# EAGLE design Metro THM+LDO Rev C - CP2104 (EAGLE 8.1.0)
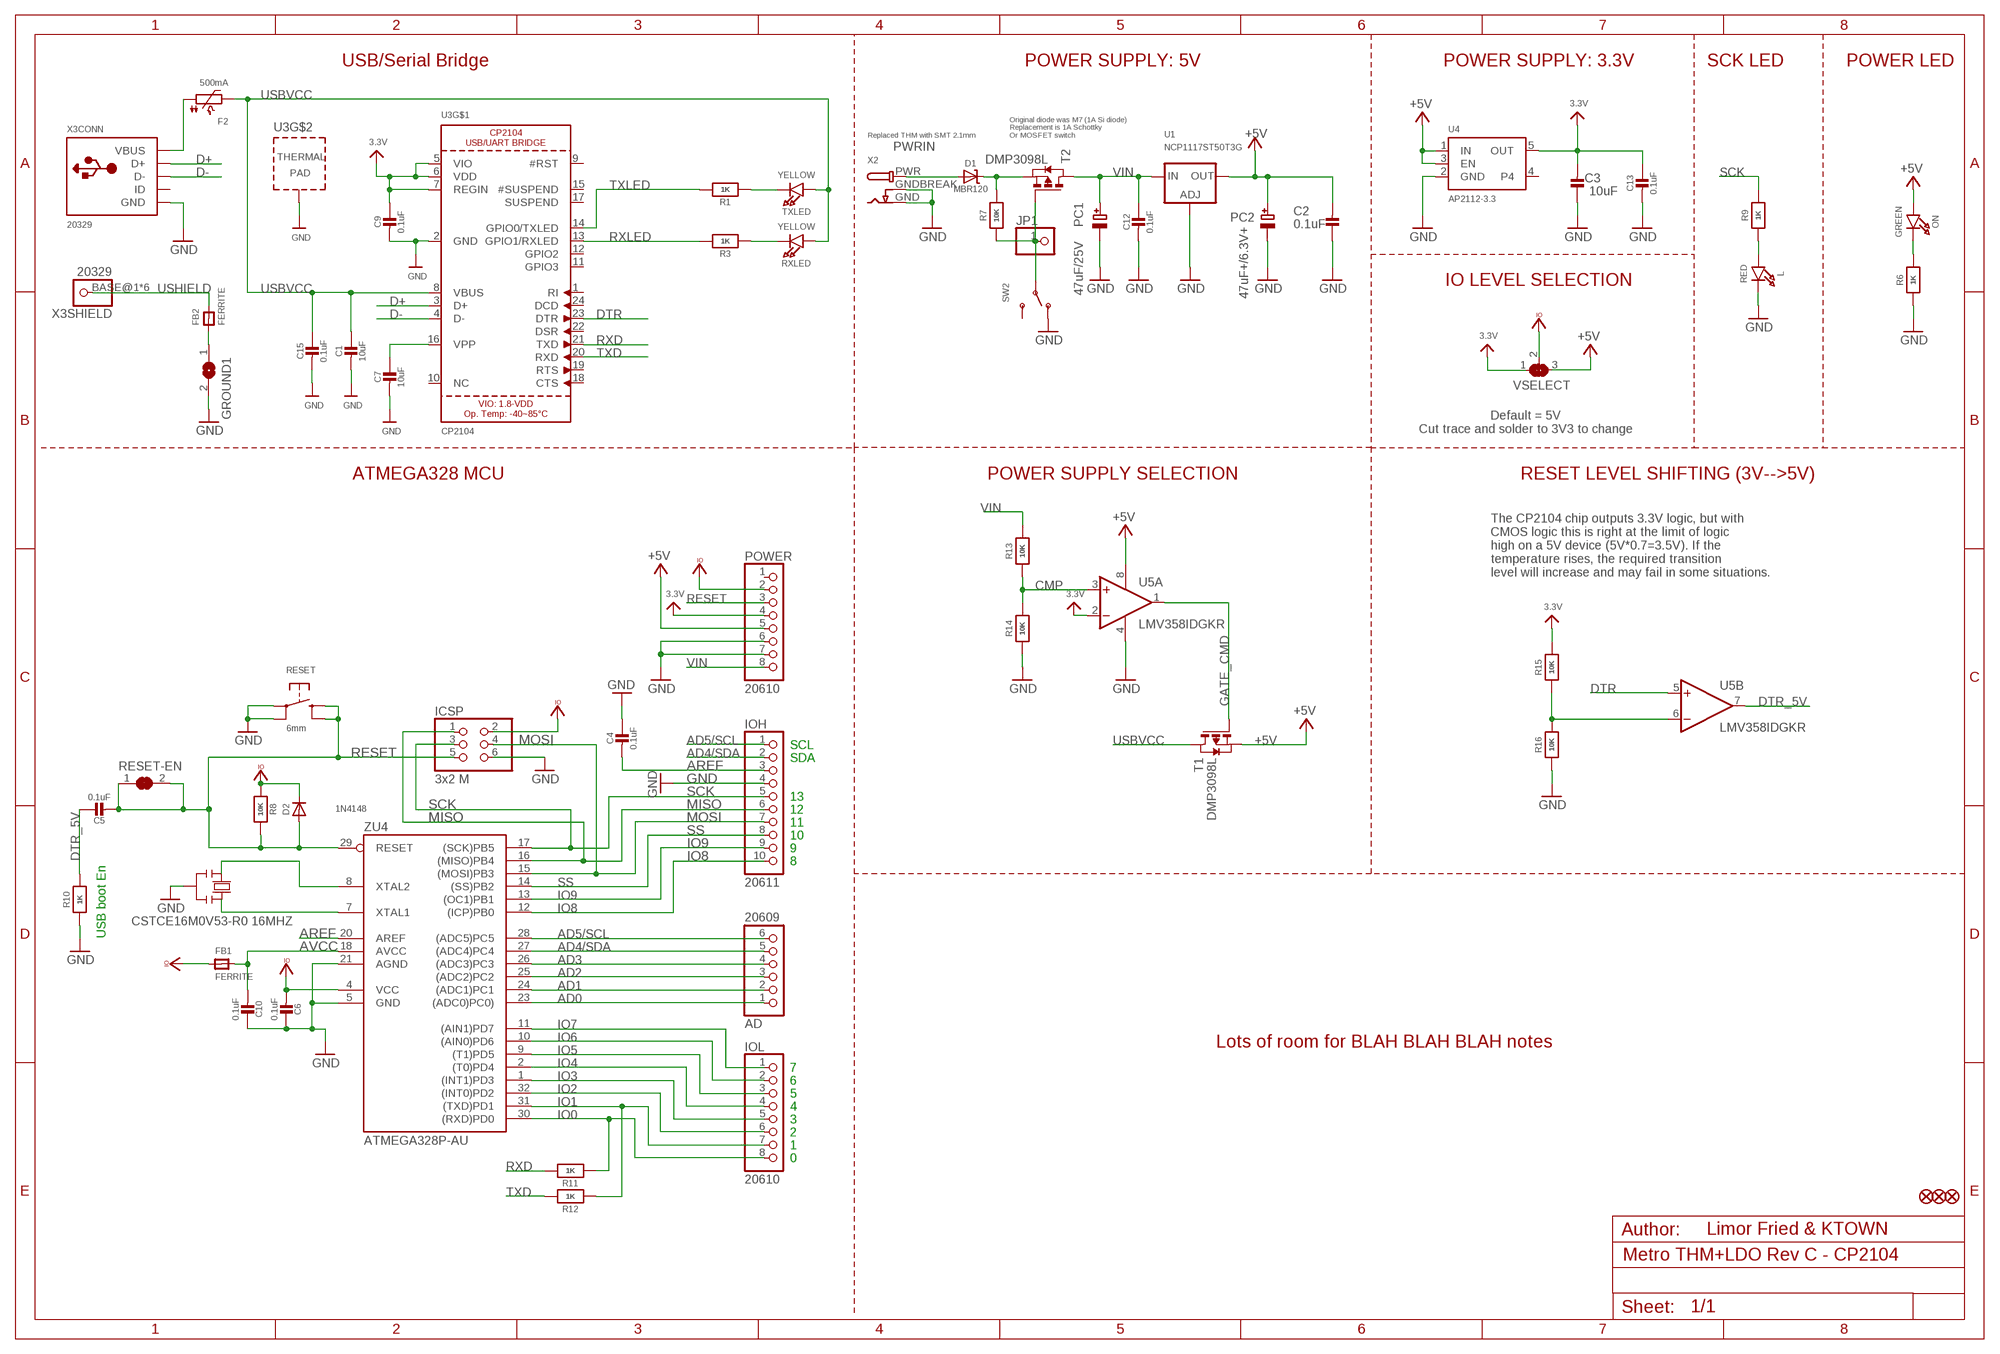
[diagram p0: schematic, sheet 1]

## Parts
AD  20609  HEADER-1X6  [1X06_OVAL]
C1  10uF  CAP_CERAMIC0805-NOOUTLINE  [0805-NO]
C2  0.1uF  CAP_CERAMIC0805-NOOUTLINE  [0805-NO]
C3  10uF  CAP_CERAMIC0805-NOOUTLINE  [0805-NO]
C4  0.1uF  CAP_CERAMIC0805-NOOUTLINE  [0805-NO]
C5  0.1uF  CAP_CERAMIC0805-NOOUTLINE  [0805-NO]
C6  0.1uF  CAP_CERAMIC0805-NOOUTLINE  [0805-NO]
C7  10uF  CAP_CERAMIC0805-NOOUTLINE  [0805-NO]
C9  0.1uF  CAP_CERAMIC0805-NOOUTLINE  [0805-NO]
C10  0.1uF  CAP_CERAMIC0805_10MGAP  [0805_10MGAP]
C12  0.1uF  CAP_CERAMIC0805-NOOUTLINE  [0805-NO]
C13  0.1uF  CAP_CERAMIC0805-NOOUTLINE  [0805-NO]
C15  0.1uF  CAP_CERAMIC0805-NOOUTLINE  [0805-NO]
D1  MBR120  DIODE-SCHOTTKYSOD-123  [SOD-123]
D2  1N4148  DIODESOD-323  [SOD-323]
F2  500mA  PTC_1206NO  [1206-NO]
FB1  FERRITE  FERRITE-0805NO  [0805-NO]
FB2  FERRITE  FERRITE-0805NO  [0805-NO]
FD1  FIDUCIAL_1MM  [FIDUCIAL_1MM]
FD2  FIDUCIAL_1MM  [FIDUCIAL_1MM]
FD3  FIDUCIAL_1MM  [FIDUCIAL_1MM]
GROUND1  SJ  [SJ]
ICSP  3x2 M  HEADER-2X3  [2X03_ROUND_70MIL]
IOH  20611  HEADER-1X10  [1X10_OVAL]
IOL  20610  HEADER-1X8  [1X08_OVAL]
JP1  HEADER-1X1ROUND  [1X01_ROUND]
L  RED  LED0805_NOOUTLINE  [CHIPLED_0805_NOOUTLINE]
ON  GREEN  LED0805_NOOUTLINE  [CHIPLED_0805_NOOUTLINE]
PC1  47uF/25V  CAP_ELECTROLYTICPANASONIC_D  [PANASONIC_D]
PC2  47uF+/6.3V+  CAP_ELECTROLYTICPANASONIC_D  [PANASONIC_D]
POWER  20610  HEADER-1X8  [1X08_OVAL]
R1  1K  RESISTOR0805_NOOUTLINE  [0805-NO]
R3  1K  RESISTOR0805_NOOUTLINE  [0805-NO]
R6  1K  RESISTOR0805_NOOUTLINE  [0805-NO]
R7  10K  RESISTOR0805_NOOUTLINE  [0805-NO]
R8  10K  RESISTOR_0805MP  [_0805MP]
R9  1K  RESISTOR0805_NOOUTLINE  [0805-NO]
R10  1K  RESISTOR0805_NOOUTLINE  [0805-NO]
R11  1K  RESISTOR0805_NOOUTLINE  [0805-NO]
R12  1K  RESISTOR0805_NOOUTLINE  [0805-NO]
R13  10K  RESISTOR0805_NOOUTLINE  [0805-NO]
R14  10K  RESISTOR0805_NOOUTLINE  [0805-NO]
R15  10K  RESISTOR0805_NOOUTLINE  [0805-NO]
R16  10K  RESISTOR0805_NOOUTLINE  [0805-NO]
RESET  6mm  SWITCH_TACT_SMT  [EVQ-Q2]
RESET-EN  SOLDERJUMPER_CLOSED  [SOLDERJUMPER_CLOSEDWIRE]
RXLED  YELLOW  LED0805_NOOUTLINE  [CHIPLED_0805_NOOUTLINE]
SW2  SWITCH_SPDT  [SPDT_SMT_SSSS811101]
T1  DMP3098L  PMOSSOT23  [SOT-23]
T2  DMP3098L  PMOSSOT23  [SOT-23]
TXLED  YELLOW  LED0805_NOOUTLINE  [CHIPLED_0805_NOOUTLINE]
U1  NCP1117ST50T3G  LM1117SOT223-REFLOW  [SOT223-R]
U3  CP2104  [QFN24_4MM_SMSC]
U4  AP2112-3.3  VREG_SOT23-5  [SOT23-5]
U5  LMV358IDGKR  LMV358MMX  [MSOP08]
VSELECT  SOLDERJUMPER_2WAY  [SOLDERJUMPER_2WAY_OPEN_NOPASTE]
X2  DCBARRELPTH  [DCJACK_2MM_PTH]
X3  20329  USB_W_SHIELD_V2  [4UCONN_20329_V2]
Y2  CSTCE16M0V53-R0 16MHZ  RESONATORMU  [RESONATOR]
ZU4  ATMEGA328P-AU  [TQFP32-08]

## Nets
3.3V: C3.2 C9.1 C13.1 POWER.4 R15.2 U3.5(VIO) U3.6(VDD) U3.7(REGIN) U4.5(OUT) U5.2(A:-IN) VSELECT.1
+5V [usbvcc]: C2.2 ON.A PC2.+ POWER.5 T1.2(S) U1.2(OUT) U1.4(OUT) U4.1(IN) U4.3(EN) U5.8(P:V+) VSELECT.3
AD0: AD.1 ZU4.23((ADC0)PC0))
AD1: AD.2 ZU4.24((ADC1)PC1)
AD2: AD.3 ZU4.25((ADC2)PC2)
AD3: AD.4 ZU4.26((ADC3)PC3)
AD4/SDA: AD.5 IOH.2 ZU4.27((ADC4)PC4)
AD5/SCL: AD.6 IOH.1 ZU4.28((ADC5)PC5)
AREF [aref]: C4.2 IOH.3 ZU4.20(AREF)
AVCC: C10.2 FB1.2 ZU4.18(AVCC)
CMP: R13.1 R14.2 U5.3(A:+IN)
D+: U3.3(D+) X3.D+(CONN:D+)
D-: U3.4(D-) X3.D-(CONN:D-)
DTR: U3.23(DTR) U5.5(B:+IN)
DTR_5V: C5.1 R10.2 U5.7(B:OUT)
GATE_CMD: T1.3(G) U5.1(A:OUT)
GND [gnd]: C1.2 C2.1 C3.1 C4.1 C6.1 C7.2 C9.2 C10.1 C12.2 C13.2 C15.2 GROUND1.2 ICSP.6 IOH.4 L.C PC1.- PC2.- POWER.6 POWER.7 R6.1 R10.1 R14.1 R16.1 RESET.A'(P1) RESET.A(P) SW2.A(O) U1.1(ADJ) U3.2(GND) U3.THERM(TP) U4.2(GND) U5.4(P:V-) X2.GND X2.GNDBREAK X3.GND(CONN:GND) Y2.2 ZU4.5(GND) ZU4.21(AGND)
IO0: IOL.8 R11.1 ZU4.30((RXD)PD0)
IO1: IOL.7 R12.1 ZU4.31((TXD)PD1)
IO2: IOL.6 ZU4.32((INT0)PD2)
IO3: IOL.5 ZU4.1((INT1)PD3)
IO4: IOL.4 ZU4.2((T0)PD4)
IO5: IOL.3 ZU4.9((T1)PD5)
IO6: IOL.2 ZU4.10((AIN0)PD6)
IO7: IOL.1 ZU4.11((AIN1)PD7)
IO8: IOH.10 ZU4.12((ICP)PB0)
IO9: IOH.9 ZU4.13((OC1)PB1)
MISO: ICSP.1 IOH.6 ZU4.16((MISO)PB4)
MOSI: ICSP.4 IOH.7 ZU4.15((MOSI)PB3)
N$1: L.A R9.1
N$2: FB2.1 GROUND1.1
N$3: ON.C R6.2
N$5: R3.1 RXLED.C
N$7: R1.1 TXLED.C
N$11: R15.1 R16.2 U5.6(B:-IN)
N$13: JP1.1 R7.1 SW2.B(P) T2.3(G)
N$15: D1.C R7.2 T2.2(S)
N$16: C7.1 U3.16(VPP)
PWRIN [power]: D1.A X2.PWR
RESET: C5.2 D2.A ICSP.5 POWER.3 R8.1 RESET-EN.1 RESET-EN.2 RESET.B'(S1) RESET.B(S) ZU4.29(RESET)
RXD: R11.2 U3.21(TXD)
RXLED: R3.2 U3.13(GPIO1/RXLED)
SCK: ICSP.3 IOH.5 R9.2 ZU4.17((SCK)PB5)
SS: IOH.8 ZU4.14((SS)PB2)
TXD: R12.2 U3.20(RXD)
TXLED: R1.2 U3.14(GPIO0/TXLED)
USBVCC [usbvcc]: C1.1 C15.1 F2.2 RXLED.A T1.1(D) TXLED.A U3.8(VBUS)
USHIELD [gnd]: FB2.2 X3.BASE@1 X3.BASE@2 X3.SPRT@1 X3.SPRT@2 X3.SPRT@3 X3.SPRT@4
VBUS: F2.1 X3.VBUS(CONN:VBUS)
VCCIO [usbvcc]: C6.2 D2.C FB1.1 ICSP.2 POWER.2 R8.2 VSELECT.2 ZU4.4(VCC)
VIN [power]: C12.1 PC1.+ POWER.8 R13.2 T2.1(D) U1.3(IN)
XTAL1: Y2.3 ZU4.7(XTAL1)
XTAL2: Y2.1 ZU4.8(XTAL2)
Unconnected: POWER.1 SW2.C(S) U3.1(RI) U3.9(#RST) U3.10(NC) U3.11(GPIO3) U3.12(GPIO2) U3.15(#SUSPEND) U3.17(SUSPEND) U3.18(CTS) U3.19(RTS) U3.22(DSR) U3.24(DCD) U4.4 X3.ID(CONN:ID)

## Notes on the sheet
- USB/Serial Bridge | POWER SUPPLY: 5V | POWER SUPPLY: 3.3V | SCK LED | POWER LED
- Replaced THM with SMT 2.1mm
- Original diode was M7 (1A Si diode)
  Replacement is 1A Schottky
  Or MOSFET switch
- IO LEVEL SELECTION
- Default = 5V
  Cut trace and solder to 3V3 to change
- ATMEGA328 MCU | POWER SUPPLY SELECTION | RESET LEVEL SHIFTING (3V-->5V)
- The CP2104 chip outputs 3.3V logic, but with
   CMOS logic this is right at the limit of logic
   high on a 5V device (5V*0.7=3.5V). If the
   temperature rises, the required transition
   level will increase and may fail in some situations.
- SCL
- SDA
- 13
- 12
- 11
- 10
- 9
- 8
- USB boot En
- Lots of room for BLAH BLAH BLAH notes
- 7
- 6
- 5
- 4
- 3
- 2
- 1
- 0
- Limor Fried & KTOWN

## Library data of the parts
AD = microbuilder:HEADER-1X6: PIN HEADER
C1-C7 C9 C10 C12 C13 C15 = microbuilder:CAP_CERAMIC: Ceramic Capacitors
D1 = microbuilder:DIODE-SCHOTTKY
D2 = microbuilder:DIODE: Diode
F2 = microbuilder:PTC: PTC (Resettable Fuse)
FB1 FB2 = microbuilder:FERRITE: Ferrite Bead
FD1-FD3 = microbuilder:FIDUCIAL: Fiducial Alignment Points; BOM: EXCLUDE
GROUND1 = jumper:SJ: SMD solder JUMPER
ICSP = microbuilder:HEADER-2X3: PIN HEADER
IOH = microbuilder:HEADER-1X10: PIN HEADER
IOL POWER = microbuilder:HEADER-1X8: PIN HEADER
JP1 = microbuilder:HEADER-1X1: PIN HEADER
L ON RXLED TXLED = microbuilder:LED: LED
PC1 PC2 = microbuilder:CAP_ELECTROLYTIC: Electrolytic Capacitors
R1 R3 R6-R16 = microbuilder:RESISTOR: Resistors
RESET = microbuilder:SWITCH_TACT_SMT: SMT Tact Switches 6x6mm - Digikey: P12940SCT-ND KMR2 (4.6x2.8mm) - Digikey: 401-1426-1-ND EVQ-PQHB55 - Light Touch, 160GF (4.5x4.5mm) - Digikey: P8090SCT-ND KMT0 - KMT021 NGJ LHS (etc.) IP68/Waterproof - Digikey: CKN10289CT-ND
RESET-EN = microbuilder:SOLDERJUMPER_CLOSED: Solder Jumper - Closed
SW2 = microbuilder:SWITCH_SPDT: Switch - SPDT SSSS811101 - Horizontal Two Position SMT, 0.3A 4V [Mouser: 688-SSSS811101]
T1 T2 = zetex:PMOSSOT23: MOS FET; OC_FARNELL: unknown; OC_NEWARK: unknown
U1 = microbuilder:LM1117: LM1117 Voltage Regulator LM1117 Adjustable Voltage regulator [Digikey: LM1117IMP-ADJDKR-ND] LM1117 3.3V Voltage regulator [AP1117E33GDIDKR-ND] LM1117 5.0V Voltage regulator [AP1117E50GDIDKR-ND] SOT223-REFLOW - SOT223 package for solder paste/reflow ovens SOT223-WAVE - SOT223 package for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
U3 = microbuilder:CP2104: CP2104 - USB to UART Bridge VDD Output: 3.45V
U4 = microbuilder:VREG_SOT23-5: SOT23-5 Fixed Voltage Regulators Part Current Out V Out V In V Dropout θJA (°C/W) TJ (°C) Digikey Part No. ADP121 150mA 3.3V 3.4-5.5V 0.09V @ 150mA -- -- ADP121-AUJZ33R7CT-ND ADP121 150mA 3.0V 3.1-5.5V 0.09V @ 150mA -- -- ADP121-AUJZ30R7CT-ND ADP122 300mA 3.3V 3.4-5.5V 0.085V @ 300mA -- --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
U5 = linear:LMV358?*: Dual General Purpose, Low Voltage, Rail-to-Rail Output Operational Amplifiers Source: http://www.national.com/mpf/LM/LMV321.html http://www.national.com/dt/lmv_qual.pdf
VSELECT = microbuilder:SOLDERJUMPER_2WAY: 2-Way Solder Jumper
X2 = microbuilder:DCBARREL: DC Barrel Jack DCJACK_1.3MM_PTH - Through Hole 1.3mm Jack (4UConnector: 05536) DCJACK_2MM_PTH - Through Hole 2.0/2.1 Jack (4UConnector: 05537) DCJACK_2MM_SMT - SMT 2.0/2.1mm Jack(4UConnector: 03267)
X3 = microbuilder:USB_W_SHIELD
Y2 = SmartPrj:RESONATOR
ZU4 = SmartPrj:ATMEGA328P-: MICROCONTROLLER 4 Kbytes FLASH 128 bytes SRAM 256 bytes EEPROM UART 6-channel 10 bit ADC

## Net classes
1 power: width 0.305 mm, drill 0.483 mm, clearance 0.203 mm
2 gnd: width 0.305 mm, drill 0.483 mm, clearance 0.203 mm
3 usbvcc: width 0.305 mm, drill 0.483 mm, clearance 0.203 mm
4 aref: width 0.254 mm, drill 0.483 mm, clearance 0.203 mm

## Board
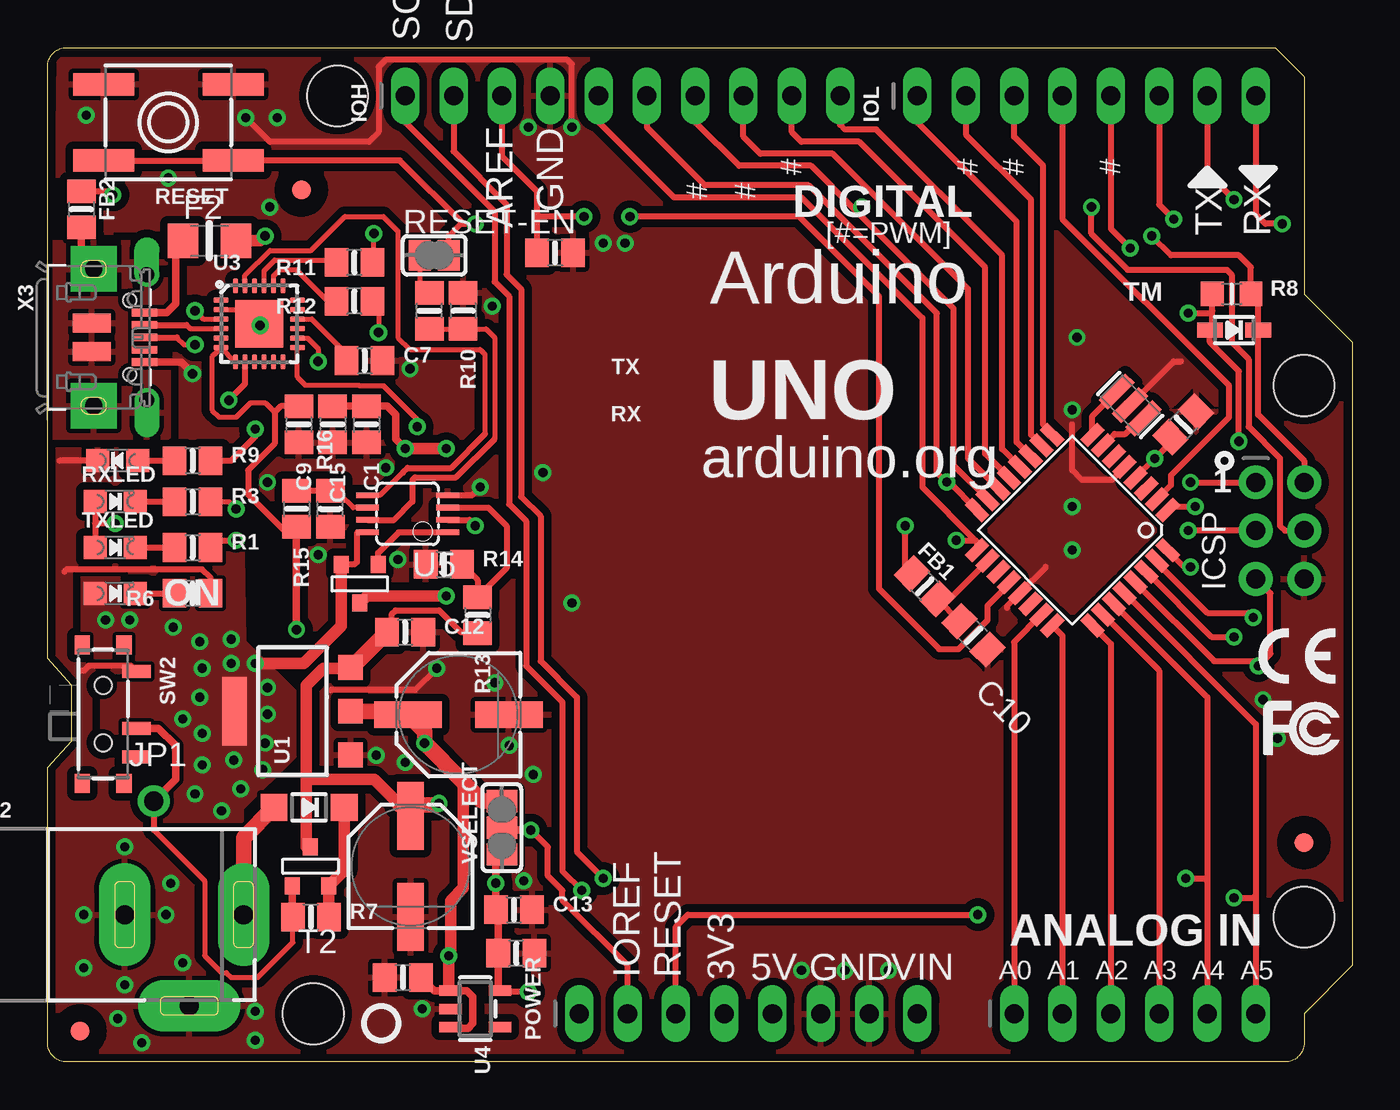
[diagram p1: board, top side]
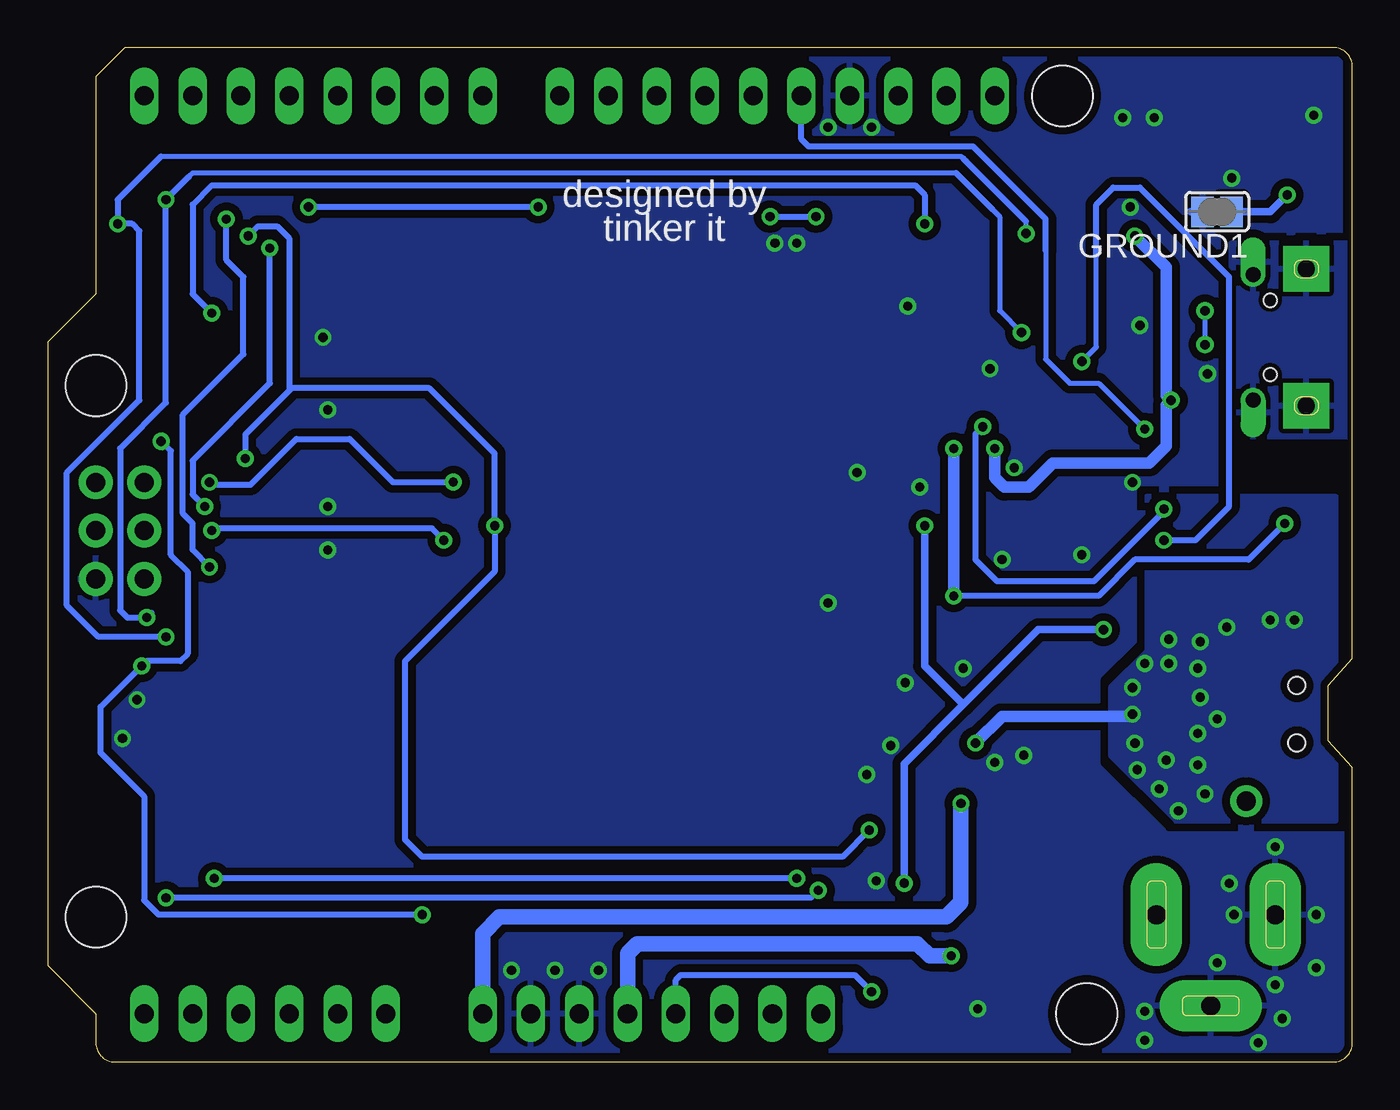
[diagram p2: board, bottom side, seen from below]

Size 68.58 x 53.34 mm. Coordinates in mm from the lower left corner, seen from the top.
Outline: 64.52,53.34 66.04,51.82 66.04,40.39 68.58,37.85 68.58,5.08 66.04,2.54 66.04,1 arc-90 65.04,0 1,0 arc-90 0,1 0,15.49 1.27,16.89 1.27,19.81 0,21.21 0,52.34 arc-90 1,53.34 64.52,53.34
Copper layers (1*16): Top 0.035mm / dielectric 1.5mm / Bottom 0.035mm
Design rules "adafruit *": minimum track width 8mil, minimum drill 15.5mil, track to track 8mil, track to pad 8mil, pad to pad 8mil, via to via 8mil, smd to smd 8mil, copper to edge 10mil, drill to drill 8mil, minimum pad ring 10mil, minimum via ring 8mil, stop-mask expansion 2mil, vias tented up to drill 20mil, thermal gap 10mil
Holes 3.2 mm at 66.04,35.56 66.04,7.62 15.24,50.8 13.97,2.54

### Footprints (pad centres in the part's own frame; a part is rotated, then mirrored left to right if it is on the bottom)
1X06_OVAL = drill 1 long: 1 -6.35,0; 2 -3.81,0; 3 -1.27,0; 4 1.27,0; 5 3.81,0; 6 6.35,0
0805-NO = smd 1.24 x 1.5: 1 -0.95,0; 2 0.95,0
0805_10MGAP = smd 1.2 x 1.5: 1 -1.05,0; 2 1.05,0
SOD-123 = smd 1.4 x 1.4: A 1.85,0; C -1.85,0
SOD-323 = smd 1.35 x 0.8: A 1.27,0; C -1.27,0
1206-NO = smd 1.6 x 1.8: 1 -1.4,0; 2 1.4,0
FIDUCIAL_1MM = smd 1 x 1: 1 0,0
SJ = smd 1.168 x 1.6: 1 -0.762,0; 2 0.762,0
2X03_ROUND_70MIL = drill 1 pad 1.778: 1 -2.54,-1.27; 2 -2.54,1.27; 3 0,-1.27; 4 0,1.27; 5 2.54,-1.27; 6 2.54,1.27
1X10_OVAL = drill 1 long: 1 -11.43,0; 2 -8.89,0; 3 -6.35,0; 4 -3.81,0; 5 -1.27,0; 6 1.27,0; 7 3.81,0; 8 6.35,0; 9 8.89,0; 10 11.43,0
1X08_OVAL = drill 1 long: 1 -8.89,0; 2 -6.35,0; 3 -3.81,0; 4 -1.27,0; 5 1.27,0; 6 3.81,0; 7 6.35,0; 8 8.89,0
1X01_ROUND = drill 1 pad 1.676: 1 0,0
CHIPLED_0805_NOOUTLINE = smd 1.2 x 1.2: A 0,-1.05; C 0,1.05
PANASONIC_D = smd 3.556 x 1.4: + 2.654,0; - -2.654,0
_0805MP = smd 1.2 x 1.3: 1 -1.016,0; 2 1.016,0
EVQ-Q2 = smd 3.2 x 1.2: A -3.4,-2; A' 3.4,-2; B -3.4,2; B' 3.4,2
SOLDERJUMPER_CLOSEDWIRE = smd 1.168 x 1.6: 1 -0.762,0; 2 0.762,0 | smd 0.635 x 0.203: WIRE 0,0
SPDT_SMT_SSSS811101 = smd 0.7 x 1.5: A -2.25,1.75; B 0.75,1.75; C 2.25,1.75 | smd 1 x 0.8: SUP1 -3.65,1.1; SUP2 -3.65,-1.1; SUP3 3.65,1.1; SUP4 3.65,-1.1 | hole 0.9: -1.5,0; 1.5,0
SOT-23 = smd 0.787 x 0.889: 1 0.025,-1.016; 2 -0.94,1.016; 3 0.991,1.016
SOT223-R = smd 1.3 x 1.3: 1 -2.3,-3.05; 2 0,-3.05; 3 2.3,-3.05 | smd 3.6 x 1.3: 4 0,3.05
QFN24_4MM_SMSC = smd 0.8 x 0.28: 1 -2,1.25; 2 -2,0.75; 3 -2,0.25; 4 -2,-0.25; 5 -2,-0.75; 6 -2,-1.25; 13 2,-1.25; 14 2,-0.75; 15 2,-0.25; 16 2,0.25; 17 2,0.75; 18 2,1.25 | smd 0.28 x 0.8: 7 -1.25,-2; 8 -0.75,-2; 9 -0.25,-2; 10 0.25,-2; 11 0.75,-2; 12 1.25,-2; 19 1.25,2; 20 0.75,2; 21 0.25,2; 22 -0.25,2; 23 -0.75,2; 24 -1.25,2 | smd 2.5 x 2.5: THERM 0,0
SOT23-5 = smd 0.55 x 1.2: 1 -0.95,-1.3; 2 0,-1.3; 3 0.95,-1.3; 4 0.95,1.3; 5 -0.95,1.3
MSOP08 = smd 0.3 x 1.2: 1 -0.976,-2.113; 2 -0.326,-2.113; 3 0.324,-2.113; 4 0.974,-2.113; 5 0.974,2.112; 6 0.324,2.112; 7 -0.326,2.112; 8 -0.976,2.112
SOLDERJUMPER_2WAY_OPEN_NOPASTE = smd 1.168 x 1.6: 1 -1.397,0; 2 0,0; 3 1.397,0
DCJACK_2MM_PTH = drill 1 pad 2.7 long: GND 7.35,0; GNDBREAK 10.75,-4.8; PWR 13.6,0
4UCONN_20329_V2 = smd 1 x 2: BASE@1 -0.75,-2; BASE@2 0.75,-2 | smd 0.4 x 1.35: D+ 0,0.775; D- -0.65,0.775; GND 1.3,0.775; ID 0.65,0.775; VBUS -1.3,0.775 | drill 0.8 pad 1.143 offset: SPRT@1 -3.3,0.9; SPRT@2 3.3,0.9 | drill 0.9 pad 2.413 square: SPRT@3 -3.6,-1.9; SPRT@4 3.6,-1.9 | hole 0.7: -1.95,0; 1.95,0
RESONATOR = smd 0.7 x 2: 1 -1,0; 2 0,0; 3 1,0
TQFP32-08 = smd 1.27 x 0.559: 1 -4.293,2.8; 2 -4.293,2; 3 -4.293,1.2; 4 -4.293,0.4; 5 -4.293,-0.4; 6 -4.293,-1.2; 7 -4.293,-2; 8 -4.293,-2.8; 17 4.293,-2.8; 18 4.293,-2; 19 4.293,-1.2; 20 4.293,-0.4; 21 4.293,0.4; 22 4.293,1.2; 23 4.293,2; 24 4.293,2.8 | smd 0.559 x 1.27: 9 -2.8,-4.293; 10 -2,-4.293; 11 -1.2,-4.293; 12 -0.4,-4.293; 13 0.4,-4.293; 14 1.2,-4.293; 15 2,-4.293; 16 2.8,-4.293; 25 2.8,4.293; 26 2,4.293; 27 1.2,4.293; 28 0.4,4.293; 29 -0.4,4.293; 30 -1.2,4.293; 31 -2,4.293; 32 -2.8,4.293

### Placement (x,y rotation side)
AD  57.15,2.54 0 top
C1  16.76,33.53 270 top
C2  18.67,4.45 0 top
C3  24.64,5.71 180 top
C4  26.67,42.55 180 top
C5  20.07,39.5 90 top
C6  59.69,33.53 225 top
C7  16.66,36.88 0 top
C9  13.21,33.53 270 top
C10  48.66,22.44 135 top
C12  18.8,22.61 0 top
C13  24.51,8 0 top
C15  14.99,33.53 270 top
D1  13.74,13.39 180 top
D2  62.36,38.48 180 top
F2  8.51,43.18 0 top
FB1  46.1,25.02 315 top
FB2  1.78,44.83 270 top
FD1  13.34,45.85 0 top
FD2  66.03,11.53 0 top
FD3  1.7,1.63 0 top
GROUND1  7.11,44.7 180 bottom
ICSP  64.77,27.94 270 top
IOH  30.23,50.8 0 top
IOL  54.61,50.8 0 top
JP1  5.59,13.72 0 top
L  3.68,31.62 90 top
ON  3.56,24.64 270 top
PC1  19.08,10.29 90 top
PC2  21.59,18.26 180 top
POWER  36.83,2.54 0 top
R1  7.62,27.05 0 top
R3  7.62,29.46 0 top
R6  7.62,24.64 180 top
R7  13.84,7.62 0 top
R8  62.23,40.39 0 top
R9  7.62,31.62 0 top
R10  21.84,39.5 270 top
R11  16.13,42.04 180 top
R12  16.13,40.01 180 top
R13  22.61,23.5 270 top
R14  20.83,26.16 0 top
R15  13.08,29.08 270 top
R16  14.86,29.08 90 top
RESET  6.35,49.4 180 top
RESET-EN  20.32,42.42 0 top
RXLED  3.56,29.46 270 top
SW2  2.92,18.29 270 top
T1  16.38,25.15 0 top
T2  13.84,10.29 180 top
TXLED  3.56,27.05 270 top
U1  12.88,18.44 90 top
U3  11.13,38.81 0 top
U4  22.48,2.79 270 top
U5  18.92,28.83 90 top
U$4  [METROSILK_CP2104_TOP]  0,0 0 top
U$14  [METROSILK_BOT]  0,0 0 top
U$15  [PCBFEAT-REV-040]  17.53,2.03 0 top
U$16  [SYMBOL_FCC_TINY]  63.91,16.15 0 top
U$17  [SYMBOL_CE_TINY]  63.65,19.91 0 top
VSELECT  23.88,12.32 90 top
X2  -3.3,7.75 0 top
X3  4.32,38.1 270 top
Y2  56.9,34.54 315 top
ZU4  53.86,27.97 225 top

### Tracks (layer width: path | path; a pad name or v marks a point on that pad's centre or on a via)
3.3V  (via drill 0.48)
  Top 0.254: U3.5 U3.6 | U3.7 U3.6 | U3.6 8.76,37.2 8.76,37.21 8.64,37.08 8.64,34.29 9.02,33.91 9.91,33.91 10.67,34.67 11.43,34.67 11.94,34.16
  Top 0.305: v25.27,3.68 23.84,3.68 | C9.1 12.25,34.48 11.94,34.16 11.94,32.51 10.54,31.11 10.54,29.84 12.45,27.94 13.02,27.94 13.02,28.07 R15.2 | U5.2 22.17,28.5 v22.48,28.19
  Top 0.406: VSELECT.1 23.56,10.61 v23.56,9.4 C13.1 23.69,7.87 C3.2 23.69,3.83 | R15.2 v13.08,22.73 | 23.69,3.83 | 23.69,3.83 U4.5 23.84,3.68 | 23.84,3.68
  Bottom 0.305: POWER.4 35.56,4.32 35.31,4.57 26.16,4.57 v25.27,3.68
  Bottom 0.406: v23.56,9.4 23.56,15.68 20.45,18.8 | 20.45,18.8 16.51,22.73 v13.08,22.73 | v22.48,28.19 22.48,20.83 20.45,18.8
+5V  (via drill 0.48)
  Top 0.305: U5.8 16.3,27.85 16.26,27.81 16.26,26.29 16.13,26.16 T1.2
  Top 0.406: C2.2 20.32,3.74 U4.1 | U4.1 22.04,3.74 22.35,3.43 22.35,2.03 22.1,1.78 21.25,1.78 U4.3 | U4.1 | U4.1 21.08,3.84
  Top 0.61: 21.84,14.69 21.84,9.14 21.18,8.48 21.18,5.68 v21.08,5.59 21.08,3.84 | T1.2 15.44,22.94 13.46,20.95 v10.92,20.95
  Top 0.813: VSELECT.3 22.82,13.72 21.84,14.69 21.84,14.73 v19.81,16.76 19.81,17.39 PC2.+ 18.76,18.44 U1.2
  Bottom 0.61: v19.81,16.76 18.41,18.16 11.81,18.16 11.68,18.29 v11.56,18.29
  Bottom 0.813: POWER.5 38.1,5.71 37.59,6.22 22.86,6.22 22.23,5.59 v21.08,5.59
  other vias: 3.05,23.24 4.32,23.24 9.65,20.95 11.56,19.68 11.43,16.76 9.78,15.88 11.3,15.37 10.16,14.35 9.65,22.23 8,22.1 8.13,20.7 8,19.18 8.13,17.27 8.13,15.62 9.14,13.21 7.75,14.1 6.6,22.86 7.11,18.03
  pour Bottom (isolate 0.406, no thermals): 0.89,29.72 10.79,29.72 10.79,21.59 12.7,19.68 12.7,16.13 9.27,12.7 0.89,12.7
  pour Top (no thermals): 1.91,12.7 1.91,14.86 2.92,15.88 2.92,20.7 1.91,21.72 1.91,29.84 10.16,29.84 10.29,22.1 12.95,19.43 12.95,16.13 10.16,13.34 10.16,12.7
AD0
  Top 0.305: ZU4.23 50.8,22.08 AD.1
AD1
  Top 0.305: ZU4.24 53.34,22.42 AD.2
AD2
  Top 0.305: ZU4.25 55.88,21.99 AD.3
AD3
  Top 0.305: ZU4.26 58.42,20.58 AD.4
AD4/SDA  (via drill 0.48)
  Top 0.305: IOH.2 21.34,47.88 24.13,45.09 24.13,41.4 24.89,40.64 24.89,29.72 25.91,28.7 25.91,21.08 27.81,19.18 27.81,11.05 v29.21,9.65 | ZU4.27 60.96,19.17 60.96,9.53 | 60.96,9.53 AD.5 | v59.82,9.65 60.83,9.65 60.96,9.53
  Bottom 0.305: v29.21,9.65 v59.82,9.65
AD5/SCL  (via drill 0.48)
  Top 0.305: ZU4.28 63.5,17.76 63.5,8.76 | IOH.1 18.8,49.4 23.5,44.7 23.5,41.02 24.26,40.26 24.26,29.34 25.15,28.45 25.15,20.83 27.05,18.92 27.05,10.03 v28.07,9.02 | 63.5,8.76 AD.6 | v62.36,8.64 63.37,8.64 63.5,8.76
  Bottom 0.305: v28.07,9.02 28.45,8.64 v62.36,8.64
AREF  (via drill 0.48)
  Top 0.305: v30.61,44.45 39.5,44.45 43.69,40.26 43.69,24.89 46.86,21.72 47.88,21.72 49.4,23.24 49.4,24 50.54,25.14 ZU4.20 | 25.72,44.45 25.72,45.78 23.88,47.62 IOH.3 | 25.72,44.45 C4.2 | v28.19,44.45 25.72,44.45
  Bottom 0.305: v30.61,44.45 v28.19,44.45
AVCC
  Top 0.305: ZU4.18 47.41,24.35 FB1.2 47.92,23.2 C10.2
CMP
  Top 0.305: U5.3 23.17,29.15 24.13,28.19 24.13,25.97 R13.1 22.61,25.33 R14.2
D+  (via drill 0.5)
  Top 0.254: 6.79,38.1 7.17,37.72 v7.75,37.72 | v7.75,39.5 8.18,39.06 U3.3
  Top 0.305: X3.D+ 6.79,38.1
  Bottom 0.254: v7.75,37.72 v7.75,39.5
D-
  Top 0.254: 7.32,38.75 7.5,38.56 U3.4
  Top 0.305: X3.D- 7.32,38.75
DTR
  Top 0.254: 22.99,33.02 22.99,37.21 22.73,37.47 19.05,37.47 18.41,38.1 18.41,43.69 17.65,44.45 15.62,44.45 13.84,42.67 11.68,42.67 10.38,41.36 U3.23 | 18.67,30.99 17.48,29.8 U5.5
  Top 0.305: 18.67,30.99 18.92,31.24 21.21,31.24 22.99,33.02
DTR_5V
  Top 0.254: 23.5,32.77 23.5,38.1 23.05,38.55 R10.2 C5.1
  Top 0.305: U5.7 18.22,28.5 19.18,29.46 19.18,30.61 19.3,30.73 21.46,30.73 23.5,32.77
GATE_CMD
  Top 0.305: U5.1 18.45,27.85 17.37,26.77 T1.3
GND  (via drill 0.48, 0.5)
  Top 0.254: U3.2 11.12,39.56 U3.THERM
  Top 0.305: Y2.2 59.18,36.83 59.56,36.83 | ZU4.5 55.93,30.61 54.36,30.61 53.85,31.11 53.85,33.53 | L.C 0.64,31.62 | 52.45,26.04 52.45,26 ZU4.21 50.42,23.96 50.42,23.88 | v27.56,49.15 27.56,52.45 27.3,52.7 17.78,52.7 17.4,52.32 17.4,48.9 16.89,48.39 11.68,48.39 v10.41,49.66 | U5.4 22.31,29.8 v22.73,30.23 | v20.45,20.7 19.3,19.56 14.86,19.56 | R6.1 8.57,25.47 8.13,25.91 1.02,25.91 0.89,25.78 | SW2.A 4.38,20.83 2.16,20.83 1.91,20.57 1.78,20.57
  Top 0.406: X3.GND 7.01,36.8 v7.62,36.2
  Bottom 0.406: GROUND1.2 8.51,44.7
  other vias: 17.78,31.24 19.68,2.79 4.06,4.06 7.11,5.21 2.03,49.78 23.5,19.94 17.27,16.13 26.04,30.99 63.88,19.05 54.1,38.1 53.85,34.29 53.85,29.21 53.85,26.92 25.02,9.53 24.26,16.64 11.68,44.96 6.35,46.48 25.27,49.15 64.64,17.02 11.56,30.48 29.21,43.05 30.35,43.05 41.91,4.83 39.62,4.83 44.2,4.83 12.06,49.66 19.05,36.45 25.53,15.11 14.22,26.67 18.41,26.42 27.56,24.13 23.37,39.75 18.8,15.75 11.18,38.73 1.91,7.75 6.22,7.75 4.06,11.3 10.92,2.67 10.92,1.14 4.95,1.02 3.68,2.29 1.91,4.95 6.48,9.4
  pour Bottom (isolate 0.406, rank 2): 0.64,52.7 67.69,52.7 67.94,52.45 67.94,0.64 0.89,0.64 0,0 0,32.38 6.86,32.26 6.73,43.56 0.64,43.69
  pour Top (isolate 0.406, rank 2): 0.64,52.7 67.94,52.7 67.94,0.64 0,0 0,32.38 6.73,32.26 6.73,43.56 0.51,43.69
IO0  (via drill 0.48, 0.5)
  Top 0.254: R11.1 17.14,42.1 v17.14,43.56
  Top 0.305: ZU4.30 61.17,22.35 v62.36,22.35 | IOL.8 63.5,44.58 64.01,44.07 v64.9,44.07
  Bottom 0.254: v17.14,43.56 17.14,44.2 | 62.61,47.62 20.57,47.62 20.32,47.37
  Bottom 0.305: v62.36,22.35 65.91,22.35 67.56,24 67.56,30.99 63.75,34.8 63.75,43.69 64.14,44.07 v64.9,44.07 64.9,45.34 62.61,47.62 | 17.14,44.2 20.32,47.37 20.45,47.5
IO1  (via drill 0.48, 0.5)
  Top 0.254: R12.1 17.4,39.69 v17.4,38.35
  Top 0.305: ZU4.31 58.31,26.27 60.96,23.62 63.12,23.62 v63.37,23.37 | IOL.7 60.96,46.74 v62.36,45.34
  Bottom 0.254: 18.92,44.83 18.54,44.45 18.54,39.5 v17.4,38.35 | 20.83,46.74 60.96,46.74 61.15,46.55
  Bottom 0.305: 18.92,44.83 20.83,46.74 | 61.15,46.55 v62.36,45.34 62.36,34.67 64.77,32.26 64.77,23.75 64.39,23.37 v63.37,23.37 63.12,23.62
IO2  (via drill 0.48)
  Top 0.305: 59.77,26.04 v60.07,26.04 59.75,26.04 ZU4.32 | v59.18,44.32 58.42,45.09 IOL.6
  Bottom 0.305: v60.07,26.04 60.96,26.92 60.96,28.32 61.47,28.83 61.47,34.04 58.29,37.21 58.29,41.27 59.18,42.16 v59.18,44.32
IO3  (via drill 0.48)
  Top 0.305: ZU4.1 59.06,29.21 v60.33,29.21 | v56.9,42.8 55.88,43.81 IOL.5
  Bottom 0.305: v56.9,42.8 56.9,35.69 60.96,31.62 60.96,29.84 v60.33,29.21
IO4
  Top 0.305: ZU4.2 59.05,30.34 59.05,30.86 62.1,33.91 62.1,35.56 53.34,44.32 IOL.4
IO5
  Top 0.305: ZU4.9 52.8,33.05 52.32,33.53 52.32,47.12 50.8,48.64 IOL.3
IO6
  Top 0.305: ZU4.10 51.69,32.97 51.69,45.34 48.26,48.77 IOL.2
IO7
  Top 0.305: ZU4.11 50.93,32.6 50.93,44.2 45.72,49.4 IOL.1
IO8
  Top 0.305: ZU4.12 50.16,32.23 50.16,42.42 43.56,49.02 41.91,49.02 41.66,49.28 IOH.10
IO9
  Top 0.305: ZU4.13 49.28,31.98 49.28,41.78 42.67,48.39 39.62,48.39 39.12,48.9 IOH.9
MISO  (via drill 0.48)
  Top 0.305: ZU4.16 47.38,30.49 v47.25,30.49 46.74,31 46.74,39.37 40.01,46.1 34.54,46.1 31.5,49.15 IOH.6 | v60.07,30.48 ICSP.1
  Bottom 0.305: v60.07,30.48 59.94,30.35 57.91,30.35 55.5,32.77 52.7,32.77 50.43,30.49 v47.25,30.49
MOSI  (via drill 0.48)
  Top 0.305: ZU4.15 47.62,31.37 47.62,39.62 42.35,44.9 | 42.35,44.9 40.13,47.12 36.34,47.12 34.04,49.42 IOH.7 | v54.86,44.96 54.86,43.56 56.77,41.66 61.98,41.66 62.23,41.4 62.23,37.85 63.12,36.96 63.12,33.4 64.77,31.75 64.77,28.19 65.02,27.94 ICSP.4 | v42.8,44.96 42.8,44.9 42.35,44.9
  Bottom 0.305: 54.99,44.96 v54.86,44.96 v42.8,44.96
N$1
  Top 0.305: L.A R9.1
N$2  (via drill 0.48)
  Top 0.305: FB2.1 3.24,45.78 v3.43,45.59
  Bottom 0.406: v3.43,45.59 4.32,44.7 GROUND1.1
N$3
  Top 0.305: ON.C R6.2
N$5
  Top 0.305: RXLED.C R3.1
N$7
  Top 0.305: TXLED.C R1.1
N$8
  Top 0.406: 23.88,13.59 23.88,12.45
N$11
  Top 0.254: U5.6 16.06,29.15 15.37,29.84 15.05,29.84 R16.2
  Top 0.305: R16.2 R15.1
N$13
  Top 0.254: 5.59,12.19 8.26,9.53 8.26,5.59 9.14,4.7 9.4,4.7 9.65,4.45 11.05,4.45 12.89,6.29 R7.1
  Top 0.305: JP1.1 5.59,12.19
  Top 0.406: R7.1 12.85,7.66 T2.3 | SW2.B 5.83,17.54 6.73,16.64 6.73,14.86 JP1.1
N$15
  Top 0.61: D1.C 15.59,10.08 T2.2 R7.2
N$16
  Top 0.254: U3.16 13.9,39.06 15.62,37.34 15.62,36.97 C7.1
PWRIN
  Top 0.813: D1.A 10.3,11.79 X2.PWR
RESET  (via drill 0.48, 0.5)
  Top 0.254: RESET-EN.1 19.56,40.95 C5.2
  Top 0.305: RESET.B' RESET.B 18.51,47.4 21.84,44.07 | ZU4.29 61.31,21.08 63.63,21.08 v63.63,20.83 64.26,21.46 64.26,24.64 ICSP.5 | v62.61,32.64 62.61,36.32 61.09,37.85 D2.A 61.21,38.61 61.21,39.5 | 61.21,39.5 R8.1 | v59.94,39.37 61.09,39.37 61.21,39.5 | POWER.3 33.02,7.11 33.66,7.75 v48.9,7.75 | 19.68,42.55 RESET-EN.1 RESET-EN.2 21.08,43.43 21.72,44.07 21.84,44.07 | v22.48,44.07 21.97,44.07 21.84,44.07
  Bottom 0.305: v59.94,39.37 60.96,40.39 60.96,45.09 59.94,46.1 22.99,46.1 22.48,45.59 v22.48,44.07 | 62.36,32.38 v62.61,32.64 62.1,32.13 62.1,26.67 61.21,25.78 61.21,21.46 61.59,21.08 63.37,21.08 v63.63,20.83 65.79,18.67 65.79,16.26 63.5,13.97 63.5,8.51 62.74,7.75 v48.9,7.75
RXD
  Top 0.254: U3.21 11.38,41.6 11.94,42.16 15.05,42.16 R11.2
RXLED  (via drill 0.48)
  Top 0.254: R3.2 9.53,29.46 v9.91,29.08 | v19.43,33.4 19.43,33.78 17.65,35.56 16.38,35.56 16.38,35.57 13.58,35.57 13.12,36.02 U3.13
  Bottom 0.305: v9.91,29.08 9.91,28.96 13.59,25.27 18.67,25.27 19.81,26.42 19.81,33.02 v19.43,33.4
SCK  (via drill 0.48)
  Top 0.305: 48.77,27.43 45.97,30.23 45.97,39.12 39.62,45.47 32.91,45.47 28.96,49.42 IOH.5 | 48.77,27.43 48.84,27.36 ZU4.17 | ICSP.3 v59.94,27.94 | v47.75,27.43 48.77,27.43 | R9.2 9.65,31.62 10.92,32.89 v10.92,33.27
  Bottom 0.254: 16.13,42.67 16.13,36.96 14.86,35.69 13.34,35.69 v10.92,33.27
  Bottom 0.305: 60.07,27.81 v59.94,27.94 59.82,28.07 48.39,28.07 v47.75,27.43 | 16.13,42.67 16.13,44.32 19.94,48.13 28.57,48.13 28.96,48.51 IOH.5
SS
  Top 0.305: ZU4.14 48.39,31.74 48.39,40.64 41.27,47.75 37.47,47.75 36.58,48.64 IOH.8
TXD
  Top 0.254: U3.20 11.88,41.34 12.19,41.66 13.08,41.66 14.73,40.01 R12.2
TXLED  (via drill 0.48, 0.5)
  Top 0.254: 8.57,27.37 R1.2 | U3.14 13.68,38.06 14.22,37.51 v14.22,36.83
  Top 0.305: 8.57,27.37 8.63,27.43 v9.91,27.43
  Bottom 0.254: 13.46,42.42 13.46,37.59 v14.22,36.83
  Bottom 0.305: 13.46,42.42 13.46,45.09 12.57,45.97 11.18,45.97 6.48,41.27 6.48,29.21 8.26,27.43 v9.91,27.43
USBVCC  (via drill 0.48, 0.5)
  Top 0.305: RXLED.A 2.51,28.32 | 2.51,28.32 TXLED.A | v3.56,28.32 2.51,28.32 | U3.8 10.38,35.65 v9.53,34.8
  Top 0.406: C15.1 C1.1 17.85,34.48 18.29,34.04 18.29,32.77 v18.8,32.26
  Top 0.61: F2.2 11.18,43.18 v11.43,43.43 | v20.95,32.26 v18.8,32.26 | v20.95,24.51 16.76,24.51 16.76,24.49 T1.1
  Bottom 0.305: v3.56,28.32 5.46,26.42 11.43,26.42 13.34,24.51 v20.95,24.51
  Bottom 0.61: v11.43,43.43 9.78,41.78 9.78,35.05 v9.53,34.8 9.78,34.54 9.78,32.38 10.67,31.5 15.75,31.5 17.02,30.23 18.29,30.23 18.8,30.73 v18.8,32.26 | v20.95,24.51 v20.95,32.26
USHIELD
  Top 0.406: FB2.2 1.78,42.34 X3.SPRT@3
  pour Bottom: 0.13,43.05 0.13,32.89 6.35,32.89 6.35,43.05
  pour Top: 0.13,43.05 0.13,32.89 6.35,32.89 6.35,43.05
VBUS
  Top 0.406: X3.VBUS 6.25,39.4 6.73,39.88 6.73,42.8 F2.1
VCCIO  (via drill 0.48)
  Top 0.305: ZU4.4 v58.19,31.73 59.02,32.56 C6.2 | FB1.1 45.09,26.04 v45.09,28.19 | v58.04,43.43 59.05,42.42 62.61,42.42 63.25,41.78 R8.2 63.63,40.01 D2.C 63.63,34.04 66.04,31.62 ICSP.2 | POWER.2 30.48,5.08 27.05,8.51 27.05,9.02 26.29,9.78 26.29,11.3 v25.4,12.19
  Top 0.406: VSELECT.2 24,12.19 v25.4,12.19
  Bottom 0.305: 55.88,35.31 55.75,35.43 48.51,35.43 45.09,32 v45.09,28.19 45.09,25.78 49.78,21.08 49.78,11.68 48.9,10.79 26.8,10.79 v25.4,12.19 | 55.88,35.31 58.19,33 v58.19,31.73 | v58.04,43.43 57.53,43.94 56.52,43.94 55.88,43.31 55.88,35.31
VIN  (via drill 0.48)
  Top 0.305: 18.1,22.55 18.1,23.56 18.29,23.75 20.57,23.75 21.72,22.61 22.35,22.61 22.67,22.61
  Top 0.406: 15.51,20.7 15.55,20.74 U1.3 | C12.1 17.91,22.55 18.1,22.55 | R13.2 22.55,22.61 22.35,22.61
  Top 0.61: 13.59,14.86 13.59,19.81 14.48,20.7 15.51,20.7 | 13.59,14.86 17.16,14.86 18.5,13.51 PC1.+ | 13.59,14.86 13.59,11.3 T2.1
  Top 0.813: v20.57,13.59 20.5,13.51 18.5,13.51 | U1.3 15.98,20.74 C12.1
  Bottom 0.813: v20.57,13.59 20.57,8.38 21.34,7.62 44.83,7.62 45.72,6.73 POWER.8
XTAL1
  Top 0.305: ZU4.7 56.08,33.02 56.64,33.02 57.46,33.84 Y2.3
XTAL2
  Top 0.305: ZU4.8 54.91,33.98 Y2.1

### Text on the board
tNames: SCL | SDA | AREF | GND | # | # | # | # | # | # | DIGITAL | [#=PWM] | TX | RX | Arduino | TM | TX | RX | UNO | arduino.org | 1 | ANALOG IN | IOREF | RESET | 3V3 | 5V | GND | VIN | A0 | A1 | A2 | A3 | A4 | A5
bNames: designed by | tinker it
214bmp: D:/SmartProjects/Snc/a4_bn_logo2.bmp

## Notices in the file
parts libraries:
microbuilder: This work is placed in the public domain, and may be freely used for commercial and non-commercial work with the following conditions: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
